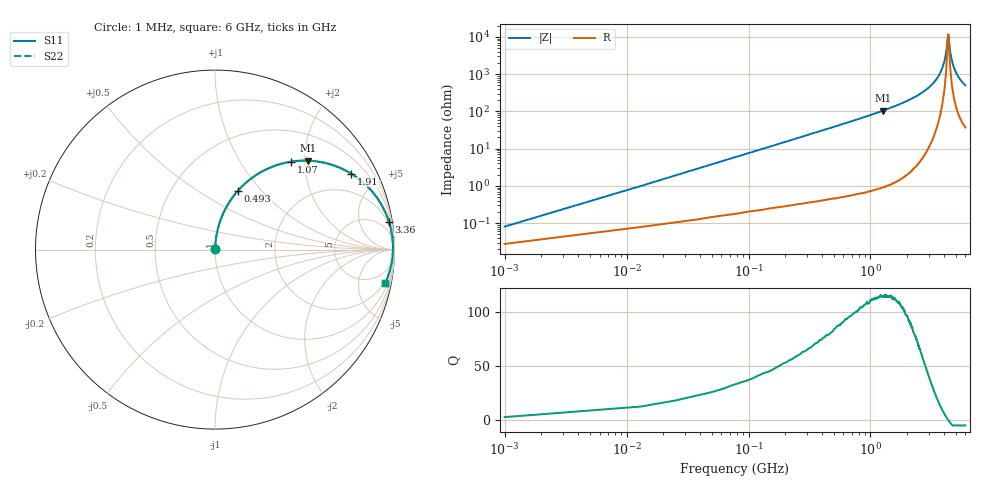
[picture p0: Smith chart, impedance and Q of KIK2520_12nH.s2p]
!version-2
!date-01.2022
!Series
# MHz S RI R 50
!Freq ReS11 ImS11 ReS21 ImS21 ReS12 ImS12 ReS22 ImS22
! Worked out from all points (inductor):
!   501 points, 1 MHz to 6 GHz, reference 50 ohm
!   read as one part in series: L = 12 nH near 25 MHz
!   highest Q = 115 at 1.26 GHz (marker M1), where L = 13.1 nH
!   self-resonance near 4.33 GHz
!   S11 on the Smith chart (normalised r, x): 1 MHz: 1.00, +0.00; 493 MHz: 1.01, +0.75; 1.07 GHz: 1.02, +1.72; 1.91 GHz: 1.04, +3.57; 3.36 GHz: 1, +13; 6 GHz: 2, -10
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1  0.000251 0.000754  0.9997 -0.000754  0.9997 -0.000754  0.000251 0.000754
37  0.00202 0.0278  0.998 -0.0278  0.998 -0.0278  0.00202 0.0278
61  0.00368 0.0458  0.9963 -0.0458  0.9963 -0.0458  0.00368 0.0458
97  0.00727 0.0725  0.9927 -0.0725  0.9927 -0.0725  0.00727 0.0725
241  0.035 0.1754  0.965 -0.1754  0.965 -0.1754  0.035 0.1754
493  0.1272 0.3272  0.8728 -0.3272  0.8728 -0.3272  0.1272 0.3272
1010  0.3937 0.4841  0.6063 -0.4841  0.6063 -0.4841  0.3937 0.4841
1070  0.4247 0.4899  0.5753 -0.4899  0.5753 -0.4899  0.4247 0.4899
1260  0.5187 0.4953  0.4813 -0.4953  0.4813 -0.4953  0.5187 0.4953
1910  0.7588 0.4229  0.2412 -0.4229  0.2412 -0.4229  0.7588 0.4229
2020  0.7875 0.4039  0.2125 -0.4039  0.2125 -0.4039  0.7875 0.4039
3010  0.9457 0.2146  0.0543 -0.2146  0.0543 -0.2146  0.9457 0.2146
3360  0.9699 0.1525  0.0301 -0.1525  0.0301 -0.1525  0.9699 0.1525
3760  0.9854 0.0868  0.0146 -0.0868  0.0146 -0.0868  0.9854 0.0868
4010  0.9901 0.048  0.00994 -0.048  0.00994 -0.048  0.9901 0.048
4180  0.9914 0.0233  0.00862 -0.0233  0.00862 -0.0233  0.9914 0.0233
4280  0.9916 0.00801  0.00844 -0.00801  0.00844 -0.00801  0.9916 0.00801
4350  0.9914 -0.000338  0.00855 0.000338  0.00855 0.000338  0.9914 -0.000338
4520  0.9903 -0.0247  0.00971 0.0247  0.00971 0.0247  0.9903 -0.0247
4640  0.9889 -0.0403  0.0111 0.0403  0.0111 0.0403  0.9889 -0.0403
5010  0.982 -0.0845  0.018 0.0845  0.018 0.0845  0.982 -0.0845
6000  0.9482 -0.1875  0.0518 0.1875  0.0518 0.1875  0.9482 -0.1875
